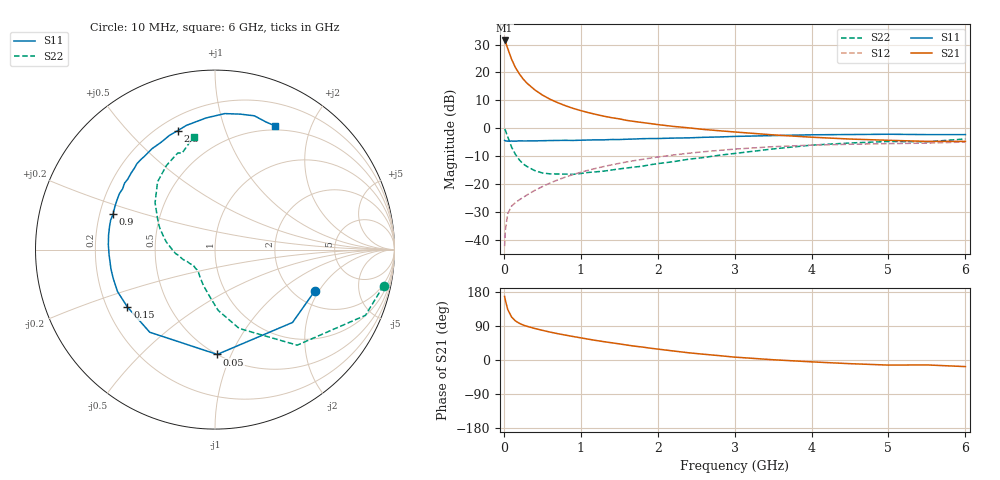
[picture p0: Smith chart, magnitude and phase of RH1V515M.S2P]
! SIEMENS Small Signal Semiconductors
! BFR106
! Si NPN RF Bipolar Junction Transistor in SOT23
! VCE = 1.5 V  IC = 15 mA
! Common Emitter S-Parameters:  August  1996
# GHz  S  MA  R  50
!  f  S11  S21  S12  S22
! GHz  MAG  ANG  MAG  ANG  MAG  ANG  MAG  ANG
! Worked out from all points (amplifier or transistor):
!   36 points, 10 MHz to 6 GHz, reference 50 ohm
!   highest |S21| = 31.5 dB at 10 MHz (marker M1)
!   |S21| within 3 dB of that: start of sweep to 51.76 MHz
!   unconditionally stable (mu >= 1): 388.5 MHz to 2.747 GHz; 4.582 GHz to end of sweep
!   at 250 MHz: K = 0.84, MSG = 21.3 dB, |S12| = -24.9 dB
!   at 1.4 GHz: K = 1.09, MAG = 6.6 dB, |S12| = -13.2 dB
!   at 6 GHz: K = 1.02, MAG = -0.8 dB, |S12| = -5.0 dB
!   S11 on the Smith chart (normalised r, x): 10 MHz: 2.57, -1.84; 50 MHz: 0.50, -0.89; 150 MHz: 0.28, -0.28; 900 MHz: 0.26, +0.16; 2.8 GHz: 0.27, +0.70; 6 GHz: 0.45, +1.50
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0.01  0.6023 -22.3  37.54 167.7  0.0076 82.2  0.9604 -12.1
0.02  0.5928 -43.2  35.66 157.5  0.0148 72.6  0.9147 -23.6
0.05  0.5842 -88.8  26.99 133.6  0.0289 55.7  0.7023 -49.3
0.1  0.5866 -128.3  17.38 113.6  0.0398 46.5  0.4592 -73.0
0.15  0.5835 -146.7  12.29 103.2  0.0459 46.5  0.3392 -87.0
0.2  0.5913 -156.7  9.502 97.0  0.0515 48.8  0.271 -95.2
0.25  0.5894 -164.4  7.652 92.4  0.057 50.5  0.228 -103.2
0.3  0.5896 -169.5  6.433 89.0  0.063 53.3  0.2051 -109.1
0.4  0.5908 -177.2  4.893 83.3  0.076 56.5  0.1732 -119.0
0.5  0.5948 177.5  3.939 78.4  0.089 58.7  0.1568 -126.0
0.6  0.5985 172.2  3.307 73.7  0.1033 59.9  0.151 -131.2
0.7  0.6015 167.7  2.869 69.5  0.1175 60.6  0.1503 -136.3
0.9  0.6014 160.7  2.268 62.0  0.1468 60.4  0.1483 -144.8
1.1  0.6119 153.1  1.898 54.9  0.1759 59.1  0.1602 -150.8
1.3  0.6162 146.6  1.64 48.4  0.2047 57.4  0.1692 -157.3
1.6  0.6325 137.7  1.377 39.4  0.2478 53.8  0.1929 -165.8
2.2  0.6627 122.0  1.076 23.9  0.3292 45.2  0.2494 176.8
2.8  0.6947 107.4  0.898 11.5  0.399 35.6  0.3265 159.5
3.5  0.7351 93.9  0.757 0.7  0.4646 24.4  0.4237 142.0
4.5  0.7678 79.4  0.637 -9.7  0.5137 9.4  0.5412 120.0
5.5  0.7658 68.3  0.579 -13.0  0.5385 0.2  0.5681 108.8
6  0.7659 64.3  0.578 -17.4  0.5633 -6.7  0.6403 100.7
